FUNCTION_BLOCK FFU
VAR_INPUT
END_VAR
VAR_OUTPUT
END_VAR
VAR
    MBMaster			:ModbusRtuMaster_KL6x22B;  // ModbusRTU Master功能块
	STAGE				:INT;
	STAGE_BF			:INT;
	
	FFU_ALARM_EN		:UINT;	//报警输出使能
	FFU_HSPEED			:UINT;	//转速上限
	FFU_LSPEED			:UINT;	//转速下限
	
	DATA_READ			:ARRAY[1..18] OF UINT;
	DATA_WRITE			:ARRAY[1..18] OF UINT;
	
	FFU_AI_STATUS		:ARRAY[1..18] OF UINT;
	FFU_AI_SPEED_PV		:ARRAY[1..18] OF UINT;
	
	FFU_AO_CTRLWORD		:ARRAY[1..3] OF UINT;
	FFU_AO_POWER_ON		:ARRAY[1..18] OF UINT;
	FFU_AO_SPEED_SV		:ARRAY[1..18] OF WORD;
	FFU_AO_EN			:ARRAY[1..18] OF UINT;
	
	FFU_CTRLWORD_BUFFER	:ARRAY[1..3] OF UINT;
	FFU_POWER_ON_BUFFER	:ARRAY[1..18] OF UINT;
	FFU_SPEED_SV_BUFFER	:ARRAY[1..18] OF UINT;
	FFU_EN_BUFFER			:ARRAY[1..18] OF UINT;
	
	WRITE_EN1			:DINT;
	WRITE_EN2			:DINT;
	WRITE_EN3			:DINT;
	WRITE_EN4			:DINT;
	WRITE_EN5			:DINT;
	WRITE_EN6			:DINT;
	WRITE_EN7			:DINT;
	
	FORCE_WRITE_TIMES	:INT;
	FORCE_WRITE			:BOOL;
	ERRID				:INT;
	TEST1:BOOL;
	TEST2:BOOL;
	TEST3:BOOL;
	TEST4:BOOL;
	TEST5:BOOL;
	TEST6:BOOL;
	TEST7:BOOL;
END_VAR

//AI数据
	AI.	FFU1_1_STATUS	:=	FFU_AI_STATUS	[	1	]	;
	AI.	FFU1_2_STATUS	:=	FFU_AI_STATUS	[	2	]	;
	AI.	FFU1_3_STATUS	:=	FFU_AI_STATUS	[	3	]	;
	AI.	FFU1_4_STATUS	:=	FFU_AI_STATUS	[	4	]	;
	AI.	FFU1_5_STATUS	:=	FFU_AI_STATUS	[	5	]	;
	AI.	FFU1_6_STATUS	:=	FFU_AI_STATUS	[	6	]	;
	AI.	FFU2_1_STATUS	:=	FFU_AI_STATUS	[	7	]	;
	AI.	FFU2_2_STATUS	:=	FFU_AI_STATUS	[	8	]	;
	AI.	FFU2_3_STATUS	:=	FFU_AI_STATUS	[	9	]	;
	AI.	FFU2_4_STATUS	:=	FFU_AI_STATUS	[	10	]	;
	AI.	FFU2_5_STATUS	:=	FFU_AI_STATUS	[	11	]	;
	AI.	FFU2_6_STATUS	:=	FFU_AI_STATUS	[	12	]	;
	AI.	FFU3_1_STATUS	:=	FFU_AI_STATUS	[	13	]	;
	AI.	FFU3_2_STATUS	:=	FFU_AI_STATUS	[	14	]	;
	AI.	FFU3_3_STATUS	:=	FFU_AI_STATUS	[	15	]	;
	AI.	FFU3_4_STATUS	:=	FFU_AI_STATUS	[	16	]	;
	AI.	FFU3_5_STATUS	:=	FFU_AI_STATUS	[	17	]	;
	AI.	FFU3_6_STATUS	:=	FFU_AI_STATUS	[	18	]	;
								
	AI.	FFU1_1_SPEED_PV	:=	FFU_AI_SPEED_PV	[	1	]	;
	AI.	FFU1_2_SPEED_PV	:=	FFU_AI_SPEED_PV	[	2	]	;
	AI.	FFU1_3_SPEED_PV	:=	FFU_AI_SPEED_PV	[	3	]	;
	AI.	FFU1_4_SPEED_PV	:=	FFU_AI_SPEED_PV	[	4	]	;
	AI.	FFU1_5_SPEED_PV	:=	FFU_AI_SPEED_PV	[	5	]	;
	AI.	FFU1_6_SPEED_PV	:=	FFU_AI_SPEED_PV	[	6	]	;
	AI.	FFU2_1_SPEED_PV	:=	FFU_AI_SPEED_PV	[	7	]	;
	AI.	FFU2_2_SPEED_PV	:=	FFU_AI_SPEED_PV	[	8	]	;
	AI.	FFU2_3_SPEED_PV	:=	FFU_AI_SPEED_PV	[	9	]	;
	AI.	FFU2_4_SPEED_PV	:=	FFU_AI_SPEED_PV	[	10	]	;
	AI.	FFU2_5_SPEED_PV	:=	FFU_AI_SPEED_PV	[	11	]	;
	AI.	FFU2_6_SPEED_PV	:=	FFU_AI_SPEED_PV	[	12	]	;
	AI.	FFU3_1_SPEED_PV	:=	FFU_AI_SPEED_PV	[	13	]	;
	AI.	FFU3_2_SPEED_PV	:=	FFU_AI_SPEED_PV	[	14	]	;
	AI.	FFU3_3_SPEED_PV	:=	FFU_AI_SPEED_PV	[	15	]	;
	AI.	FFU3_4_SPEED_PV	:=	FFU_AI_SPEED_PV	[	16	]	;
	AI.	FFU3_5_SPEED_PV	:=	FFU_AI_SPEED_PV	[	17	]	;
	AI.	FFU3_6_SPEED_PV	:=	FFU_AI_SPEED_PV	[	18	]	;

//AO数据比较
	FFU_AO_CTRLWORD	[	1	]	:=	AO.	FFU_ALARM_EN	;
	FFU_AO_CTRLWORD	[	2	]	:=	AO.	FFU_LSPEED		;
	FFU_AO_CTRLWORD	[	3	]	:=	AO.	FFU_HSPEED	;
								
	FFU_AO_POWER_ON	[	1	]	:=	AO.	FFU1_1_POWER_ON	;
	FFU_AO_POWER_ON	[	2	]	:=	AO.	FFU1_2_POWER_ON	;
	FFU_AO_POWER_ON	[	3	]	:=	AO.	FFU1_3_POWER_ON	;
	FFU_AO_POWER_ON	[	4	]	:=	AO.	FFU1_4_POWER_ON	;
	FFU_AO_POWER_ON	[	5	]	:=	AO.	FFU1_5_POWER_ON	;
	FFU_AO_POWER_ON	[	6	]	:=	AO.	FFU1_6_POWER_ON	;
	FFU_AO_POWER_ON	[	7	]	:=	AO.	FFU2_1_POWER_ON	;
	FFU_AO_POWER_ON	[	8	]	:=	AO.	FFU2_2_POWER_ON	;
	FFU_AO_POWER_ON	[	9	]	:=	AO.	FFU2_3_POWER_ON	;
	FFU_AO_POWER_ON	[	10	]	:=	AO.	FFU2_4_POWER_ON	;
	FFU_AO_POWER_ON	[	11	]	:=	AO.	FFU2_5_POWER_ON	;
	FFU_AO_POWER_ON	[	12	]	:=	AO.	FFU2_6_POWER_ON	;
	FFU_AO_POWER_ON	[	13	]	:=	AO.	FFU3_1_POWER_ON	;
	FFU_AO_POWER_ON	[	14	]	:=	AO.	FFU3_2_POWER_ON	;
	FFU_AO_POWER_ON	[	15	]	:=	AO.	FFU3_3_POWER_ON	;
	FFU_AO_POWER_ON	[	16	]	:=	AO.	FFU3_4_POWER_ON	;
	FFU_AO_POWER_ON	[	17	]	:=	AO.	FFU3_5_POWER_ON	;
	FFU_AO_POWER_ON	[	18	]	:=	AO.	FFU3_6_POWER_ON	;
								
	FFU_AO_SPEED_SV	[	1	]	:=	AO.	FFU1_1_SPEED_SV	;
	FFU_AO_SPEED_SV	[	2	]	:=	AO.	FFU1_2_SPEED_SV	;
	FFU_AO_SPEED_SV	[	3	]	:=	AO.	FFU1_3_SPEED_SV	;
	FFU_AO_SPEED_SV	[	4	]	:=	AO.	FFU1_4_SPEED_SV	;
	FFU_AO_SPEED_SV	[	5	]	:=	AO.	FFU1_5_SPEED_SV	;
	FFU_AO_SPEED_SV	[	6	]	:=	AO.	FFU1_6_SPEED_SV	;
	FFU_AO_SPEED_SV	[	7	]	:=	AO.	FFU2_1_SPEED_SV	;
	FFU_AO_SPEED_SV	[	8	]	:=	AO.	FFU2_2_SPEED_SV	;
	FFU_AO_SPEED_SV	[	9	]	:=	AO.	FFU2_3_SPEED_SV	;
	FFU_AO_SPEED_SV	[	10	]	:=	AO.	FFU2_4_SPEED_SV	;	
	FFU_AO_SPEED_SV	[	11	]	:=	AO.	FFU2_5_SPEED_SV	;
	FFU_AO_SPEED_SV	[	12	]	:=	AO.	FFU2_6_SPEED_SV	;
	FFU_AO_SPEED_SV	[	13	]	:=	AO.	FFU3_1_SPEED_SV	;
	FFU_AO_SPEED_SV	[	14	]	:=	AO.	FFU3_2_SPEED_SV	;
	FFU_AO_SPEED_SV	[	15	]	:=	AO.	FFU3_3_SPEED_SV	;
	FFU_AO_SPEED_SV	[	16	]	:=	AO.	FFU3_4_SPEED_SV	;
	FFU_AO_SPEED_SV	[	17	]	:=	AO.	FFU3_5_SPEED_SV	;
	FFU_AO_SPEED_SV	[	18	]	:=	AO.	FFU3_6_SPEED_SV	;
	
	FFU_AO_EN	[	1	]	:=	AO.	FFU1_1_EN	;
	FFU_AO_EN	[	2	]	:=	AO.	FFU1_2_EN	;
	FFU_AO_EN	[	3	]	:=	AO.	FFU1_3_EN	;
	FFU_AO_EN	[	4	]	:=	AO.	FFU1_4_EN	;
	FFU_AO_EN	[	5	]	:=	AO.	FFU1_5_EN	;
	FFU_AO_EN	[	6	]	:=	AO.	FFU1_6_EN	;
	FFU_AO_EN	[	7	]	:=	AO.	FFU2_1_EN	;
	FFU_AO_EN	[	8	]	:=	AO.	FFU2_2_EN	;
	FFU_AO_EN	[	9	]	:=	AO.	FFU2_3_EN	;
	FFU_AO_EN	[	10	]	:=	AO.	FFU2_4_EN	;	
	FFU_AO_EN	[	11	]	:=	AO.	FFU2_5_EN	;
	FFU_AO_EN	[	12	]	:=	AO.	FFU2_6_EN	;
	FFU_AO_EN	[	13	]	:=	AO.	FFU3_1_EN	;
	FFU_AO_EN	[	14	]	:=	AO.	FFU3_2_EN	;
	FFU_AO_EN	[	15	]	:=	AO.	FFU3_3_EN	;
	FFU_AO_EN	[	16	]	:=	AO.	FFU3_4_EN	;
	FFU_AO_EN	[	17	]	:=	AO.	FFU3_5_EN	;
	FFU_AO_EN	[	18	]	:=	AO.	FFU3_6_EN	;



	WRITE_EN1:=MEMCMP(pBuf1:=ADR(FFU_AO_CTRLWORD) , pBuf2:= ADR(FFU_CTRLWORD_BUFFER), n:=SIZEOF(FFU_CTRLWORD_BUFFER) );
	
	WRITE_EN2:=MEMCMP(pBuf1:=ADR(FFU_AO_POWER_ON) , pBuf2:= ADR(FFU_POWER_ON_BUFFER), n:=SIZEOF(FFU_POWER_ON_BUFFER) );
	
	WRITE_EN3:=MEMCMP(pBuf1:=ADR(FFU_AO_SPEED_SV) , pBuf2:= ADR(FFU_SPEED_SV_BUFFER), n:=SIZEOF(FFU_SPEED_SV_BUFFER) );
	
	WRITE_EN4:=MEMCMP(pBuf1:=ADR(FFU_AO_EN) , pBuf2:= ADR(FFU_EN_BUFFER), n:=SIZEOF(FFU_EN_BUFFER) );
	
	
	
IF FORCE_WRITE_TIMES>=1000 
	THEN 
	FORCE_WRITE:=TRUE;	
END_IF


(*
	MBMaster.WriteRegs(
	UnitID:= 1, 
	Quantity:= 18, 
	MBAddr:= 16#401, 
	cbLength:= SIZEOF(FFU_AO_SPEED_SV), 
	pMemoryAddr:= ADR(FFU_AO_SPEED_SV), 
	Execute:= TEST6,//TRUE, 
	Timeout:= T#2000MS,
	);
	TEST6:=FALSE;
	MBMaster.BUSY;
	MBMaster.Error;
	MBMaster.ErrorId;
*)
(*
	MBMaster.ReadRegs(
	UnitID:= 1, 
	Quantity:= 18, 
	MBAddr:= 257, 
	cbLength:= SIZEOF(FFU_AI_STATUS), 
	pMemoryAddr:= ADR(FFU_AI_STATUS), 
	Execute:= TEST1,//TRUE, 
	Timeout:= T#200MS, 
	 );
	ERRID:= MBMaster.ErrorId;
	IF NOT MBMaster.BUSY THEN
		TEST1:=FALSE; 
		//MBMaster.ReadRegs(Execute:=FALSE,);
		//FORCE_WRITE_TIMES:=FORCE_WRITE_TIMES+1;
		STAGE:=2;
	END_IF
*)

CASE STAGE OF 
	0://首次通讯
	STAGE:=1;
	
	1://读状态
	MBMaster.ReadRegs(
	UnitID:= 1, 
	Quantity:= 18, 
	MBAddr:= 257, 
	cbLength:= SIZEOF(FFU_AI_STATUS), 
	pMemoryAddr:= ADR(FFU_AI_STATUS), 
	Execute:= TRUE, 
	Timeout:= T#200MS, 
	 );
	IF NOT MBMaster.BUSY THEN
		//TEST1:=FALSE; 
		MBMaster.ReadRegs(Execute:=FALSE,);
		FORCE_WRITE_TIMES:=FORCE_WRITE_TIMES+1;
		STAGE:=2;
	END_IF
	
	2://读转速
	MBMaster.ReadRegs(
	UnitID:= 1, 
	Quantity:= 18, 
	MBAddr:= 513, 
	cbLength:= SIZEOF(FFU_AI_SPEED_PV), 
	pMemoryAddr:= ADR(FFU_AI_SPEED_PV), 
	Execute:= TRUE, 
	Timeout:= T#200MS, 
	 );
	IF NOT MBMaster.BUSY THEN
		//TEST2:=FALSE; 
		MBMaster.ReadRegs(Execute:=FALSE,);
		FORCE_WRITE_TIMES:=FORCE_WRITE_TIMES+1;
		STAGE:=3;
	END_IF
	
	3://数值变更判断
	IF WRITE_EN1<>0 OR FORCE_WRITE
		THEN
		STAGE:=4;
		ELSIF WRITE_EN2<>0
			THEN
			STAGE:=5;
			ELSIF WRITE_EN3<>0
				THEN
				STAGE:=6;
				ELSIF WRITE_EN4<>0
					THEN
					STAGE:=7;
					ELSIF WRITE_EN5<>0
						THEN
						STAGE:=8;				
	ELSE
		STAGE:=1;
	END_IF
	
	4://写控制字
	MBMaster.WriteRegs(
	UnitID:= 1, 
	Quantity:= 3, 
	MBAddr:= 2, 
	cbLength:= SIZEOF(FFU_AO_CTRLWORD), 
	pMemoryAddr:= ADR(FFU_AO_CTRLWORD), 
	Execute:= TRUE, 
	Timeout:= T#200MS,
	);
	IF NOT MBMaster.BUSY THEN 
		//TEST4:=FALSE;
		MBMaster.WriteRegs(Execute:=FALSE,);
		MEMCPY(destAddr:= ADR(FFU_CTRLWORD_BUFFER), srcAddr:= ADR(FFU_AO_CTRLWORD), n:= SIZEOF(FFU_AO_CTRLWORD));
		IF NOT FORCE_WRITE
		THEN
		STAGE:=1;
		ELSE
		STAGE:=5;
		END_IF		
	END_IF
	
	5://写启停
	MBMaster.WriteRegs(
	UnitID:= 1, 
	Quantity:= 18, 
	MBAddr:= 769, 
	cbLength:= SIZEOF(FFU_AO_POWER_ON), 
	pMemoryAddr:= ADR(FFU_AO_POWER_ON), 
	Execute:= TRUE, 
	Timeout:= T#200MS,
	);
	IF NOT MBMaster.BUSY THEN 
		//TEST5:=FALSE;
		MBMaster.WriteRegs(Execute:=FALSE,);
		MEMCPY(destAddr:= ADR(FFU_POWER_ON_BUFFER), srcAddr:= ADR(FFU_AO_POWER_ON), n:= SIZEOF(FFU_AO_POWER_ON));
		IF NOT FORCE_WRITE
		THEN
		STAGE:=1;
		ELSE
		STAGE:=6;
		END_IF		
	END_IF
	
	6://写转速
	MBMaster.WriteRegs(
	UnitID:= 1, 
	Quantity:= 18, 
	MBAddr:= 1025, 
	cbLength:= SIZEOF(FFU_AO_SPEED_SV), 
	pMemoryAddr:= ADR(FFU_AO_SPEED_SV), 
	Execute:= TRUE, 
	Timeout:= T#200MS,
	);
	IF NOT MBMaster.BUSY THEN 
		//TEST6:=FALSE;
		MBMaster.WriteRegs(Execute:=FALSE,);
		MEMCPY(destAddr:= ADR(FFU_SPEED_SV_BUFFER), srcAddr:= ADR(FFU_AO_SPEED_SV), n:= SIZEOF(FFU_AO_SPEED_SV));
		IF NOT FORCE_WRITE
		THEN
		STAGE:=1;
		ELSE
		STAGE:=7;
		END_IF		
	END_IF
	
	7://写使能
	MBMaster.WriteRegs(
	UnitID:= 1, 
	Quantity:= 18, 
	MBAddr:= 1281, 
	cbLength:= SIZEOF(FFU_AO_EN), 
	pMemoryAddr:= ADR(FFU_AO_EN), 
	Execute:= TRUE, 
	Timeout:= T#200MS,
	);
	IF NOT MBMaster.BUSY THEN 
		//TEST7:=FALSE;
		MBMaster.WriteRegs(Execute:=FALSE,);
		MEMCPY(destAddr:= ADR(FFU_EN_BUFFER), srcAddr:= ADR(FFU_AO_EN), n:= SIZEOF(FFU_AO_EN));
		STAGE:=1;
		IF FORCE_WRITE
		THEN
		FORCE_WRITE_TIMES:=0;
		FORCE_WRITE:=FALSE;
		END_IF		
	END_IF	
END_CASE

END_FUNCTION_BLOCK
